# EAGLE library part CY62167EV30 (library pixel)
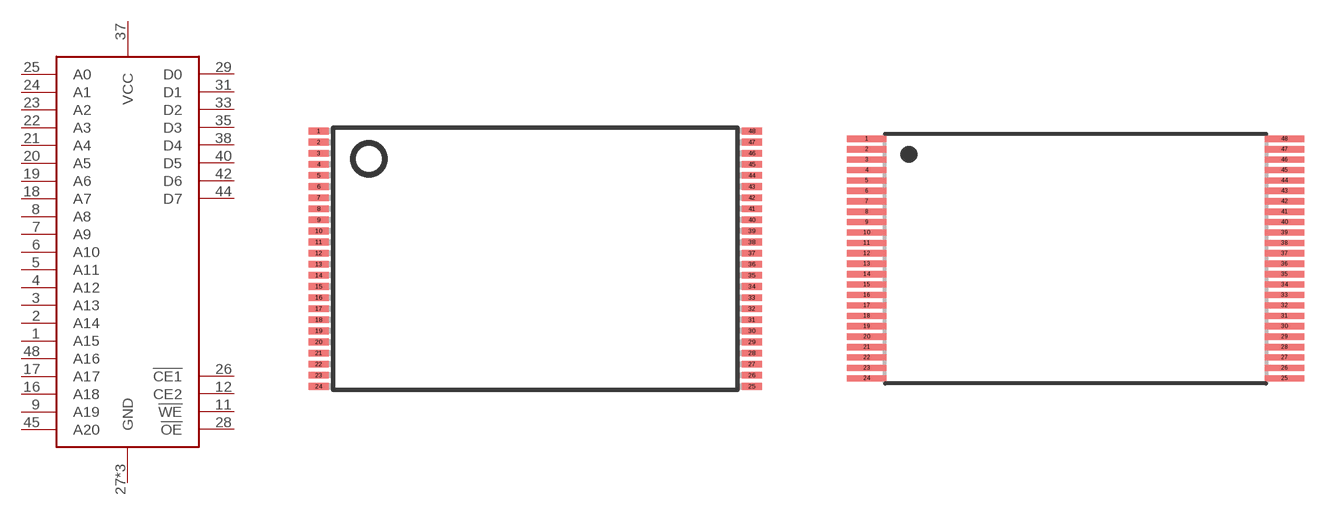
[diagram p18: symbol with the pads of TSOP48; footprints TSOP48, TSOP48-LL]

Designator prefix -

## CY62167EV30  [TSOP48]
1  A15
2  A14
3  A13
4  A12
5  A11
6  A10
7  A9
8  A8
9  A19
11  !WE
12  CE2
16  A18
17  A17
18  A7
19  A6
20  A5
21  A4
22  A3
23  A2
24  A1
25  A0
26  !CE1
27  GND
28  !OE
29  D0
31  D1
33  D2
35  D3
37  VCC
38  D4
40  D5
42  D6
44  D7
45  A20
46  GND
47  GND
48  A16

## CY62167EV30LL  [TSOP48-LL]
Pads as for TSOP48

## Footprint TSOP48 (pad centres in mm)
48-Pin TSOP OCPL Type 1 (WC Package Code) Source: http://download.micron.com/pdf/datasheets/flash/nand/4gb_nand_m40a.pdf
smd 0.9 x 0.3: 1 -9.75,5.75; 2 -9.75,5.25; 3 -9.75,4.75; 4 -9.75,4.25; 5 -9.75,3.75; 6 -9.75,3.25; 7 -9.75,2.75; 8 -9.75,2.25; 9 -9.75,1.75; 10 -9.75,1.25; 11 -9.75,0.75; 12 -9.75,0.25; 13 -9.75,-0.25; 14 -9.75,-0.75; 15 -9.75,-1.25; 16 -9.75,-1.75; 17 -9.75,-2.25; 18 -9.75,-2.75; 19 -9.75,-3.25; 20 -9.75,-3.75; 21 -9.75,-4.25; 22 -9.75,-4.75; 23 -9.75,-5.25; 24 -9.75,-5.75; 25 9.75,-5.75; 26 9.75,-5.25; 27 9.75,-4.75; 28 9.75,-4.25; 29 9.75,-3.75; 30 9.75,-3.25; 31 9.75,-2.75; 32 9.75,-2.25; 33 9.75,-1.75; 34 9.75,-1.25; 35 9.75,-0.75; 36 9.75,-0.25; 37 9.75,0.25; 38 9.75,0.75; 39 9.75,1.25; 40 9.75,1.75; 41 9.75,2.25; 42 9.75,2.75; 43 9.75,3.25; 44 9.75,3.75; 45 9.75,4.25; 46 9.75,4.75; 47 9.75,5.25; 48 9.75,5.75

## Footprint TSOP48-LL (pad centres in mm)
48-Lead Thin Small Outline Package (TSOP) 12mm x 20mm SST Package Code: EK Source: http://www.sst.com/dotAsset/40687.pdf
smd 1.9 x 0.3: 1 -10.025,5.75; 2 -10.025,5.25; 3 -10.025,4.75; 4 -10.025,4.25; 5 -10.025,3.75; 6 -10.025,3.25; 7 -10.025,2.75; 8 -10.025,2.25; 9 -10.025,1.75; 10 -10.025,1.25; 11 -10.025,0.75; 12 -10.025,0.25; 13 -10.025,-0.25; 14 -10.025,-0.75; 15 -10.025,-1.25; 16 -10.025,-1.75; 17 -10.025,-2.25; 18 -10.025,-2.75; 19 -10.025,-3.25; 20 -10.025,-3.75; 21 -10.025,-4.25; 22 -10.025,-4.75; 23 -10.025,-5.25; 24 -10.025,-5.75; 25 10.025,-5.75; 26 10.025,-5.25; 27 10.025,-4.75; 28 10.025,-4.25; 29 10.025,-3.75; 30 10.025,-3.25; 31 10.025,-2.75; 32 10.025,-2.25; 33 10.025,-1.75; 34 10.025,-1.25; 35 10.025,-0.75; 36 10.025,-0.25; 37 10.025,0.25; 38 10.025,0.75; 39 10.025,1.25; 40 10.025,1.75; 41 10.025,2.25; 42 10.025,2.75; 43 10.025,3.25; 44 10.025,3.75; 45 10.025,4.25; 46 10.025,4.75; 47 10.025,5.25; 48 10.025,5.75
